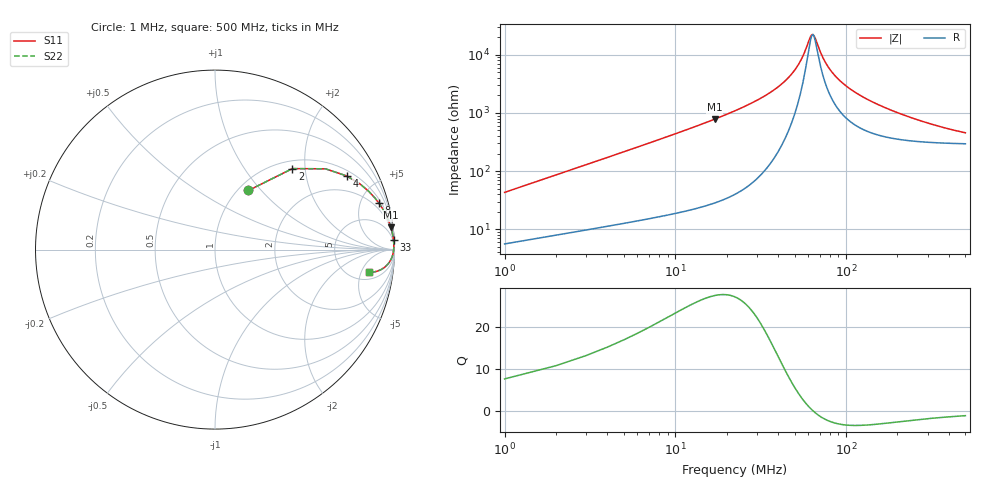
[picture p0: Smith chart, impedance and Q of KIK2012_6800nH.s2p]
!version-2
!date-01.2022
!Series
# MHz S RI R 50
!Freq ReS11 ImS11 ReS21 ImS21 ReS12 ImS12 ReS22 ImS22
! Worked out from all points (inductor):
!   500 points, 1 MHz to 500 MHz, reference 50 ohm
!   read as one part in series: L = 6.8 uH near 3 MHz
!   highest Q = 27.4 at 17 MHz (marker M1), where L = 7.32 uH
!   self-resonance near 63 MHz
!   S11 on the Smith chart (normalised r, x): 1 MHz: 1.11, +0.85; 2 MHz: 1.16, +1.71; 4 MHz: 1.22, +3.43; 8 MHz: 1.33, +6.95; 33 MHz: 3, +38; 500 MHz: 6.91, -6.95
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1  0.1863 0.3293  0.8137 -0.3293  0.8137 -0.3293  0.1863 0.3293
2  0.4309 0.4511  0.5691 -0.4511  0.5691 -0.4511  0.4309 0.4511
4  0.734 0.4103  0.266 -0.4103  0.266 -0.4103  0.734 0.4103
6  0.8574 0.3238  0.1426 -0.3238  0.1426 -0.3238  0.8574 0.3238
8  0.9133 0.2589  0.0867 -0.2589  0.0867 -0.2589  0.9133 0.2589
17  0.9796 0.1245  0.0204 -0.1245  0.0204 -0.1245  0.9796 0.1245
33  0.9947 0.0515  0.0053 -0.0515  0.0053 -0.0515  0.9947 0.0515
50  0.9965 0.018  0.00355 -0.018  0.00355 -0.018  0.9965 0.018
55  0.9963 0.0109  0.00372 -0.0109  0.00372 -0.0109  0.9963 0.0109
61  0.9958 0.00342  0.00415 -0.00342  0.00415 -0.00342  0.9958 0.00342
63  0.9957 0.0011  0.00434 -0.0011  0.00434 -0.0011  0.9957 0.0011
66  0.9953 -0.00223  0.00466 0.00223  0.00466 0.00223  0.9953 -0.00223
72  0.9946 -0.00845  0.00543 0.00845  0.00543 0.00845  0.9946 -0.00845
76  0.994 -0.0123  0.00601 0.0123  0.00601 0.0123  0.994 -0.0123
85  0.9925 -0.0204  0.00753 0.0204  0.00753 0.0204  0.9925 -0.0204
98  0.9899 -0.0307  0.0101 0.0307  0.0101 0.0307  0.9899 -0.0307
116  0.9856 -0.0433  0.0144 0.0433  0.0144 0.0433  0.9856 -0.0433
168  0.9701 -0.0721  0.0299 0.0721  0.0299 0.0721  0.9701 -0.0721
251  0.9399 -0.1023  0.0601 0.1023  0.0601 0.1023  0.9399 -0.1023
334  0.909 -0.1184  0.091 0.1184  0.091 0.1184  0.909 -0.1184
417  0.881 -0.1249  0.119 0.1249  0.119 0.1249  0.881 -0.1249
500  0.8573 -0.1254  0.1427 0.1254  0.1427 0.1254  0.8573 -0.1254
